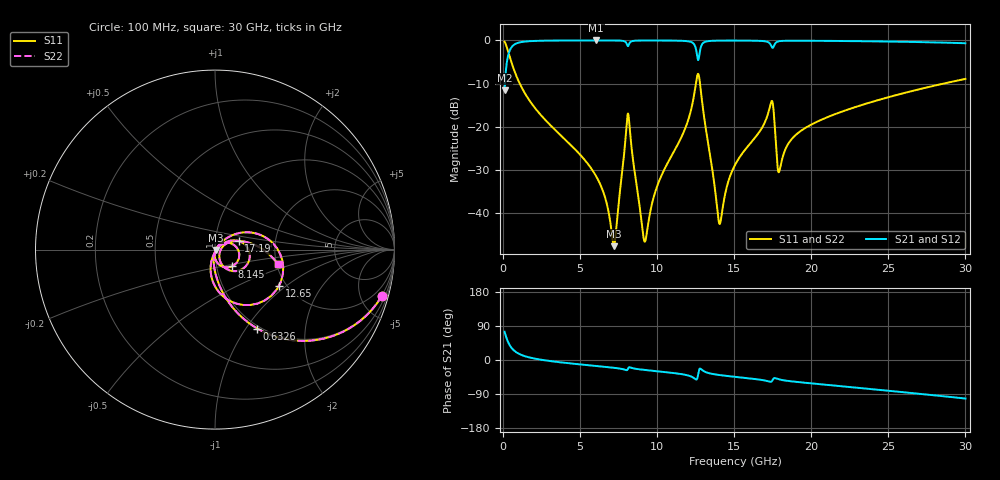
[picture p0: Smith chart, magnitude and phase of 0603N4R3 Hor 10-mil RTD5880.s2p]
# GHz S MA R 50
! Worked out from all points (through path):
!   3201 points, 100 MHz to 30 GHz, reference 50 ohm
!   highest |S21| = -0.03 dB at 6.043 GHz (marker M1); lowest = -11.6 dB at 100 MHz (marker M2)
!   group delay of S21, straight-line fit = 10.4 ps
!   lowest |S11| = -47.6 dB at 7.192 GHz (marker M3), VSWR 1.01, Z = 50.4 - j0.192 ohm
!   |S11| at or under -10 dB: 1.082 GHz to 12.51 GHz (11.43 GHz wide, 168 % of centre); 12.78 GHz to 28.58 GHz (15.8 GHz wide, 76.4 % of centre)
!   |S22| runs from -47.6 to -0.3 dB; largest |S21 - S12| = 0
!   S11 on the Smith chart (normalised r, x): 100 MHz: 0.97, -7.19; 632.6 MHz: 0.97, -1.13; 8.145 GHz: 1.19, -0.23; 12.65 GHz: 1.83, -0.89; 17.19 GHz: 1.30, +0.13; 30 GHz: 2.03, -0.37
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0.1  0.9646 -15.6  0.2635 74.4  0.2635 74.4  0.9646 -15.6
0.6325937  0.4988 -61.8  0.866 28.1  0.866 28.1  0.4988 -61.8
1.66975  0.207 -82.5  0.9771 7.1  0.9771 7.1  0.207 -82.5
5.089563  0.04575 -99.1  0.9965 -12.0  0.9965 -12.0  0.04575 -99.1
6.042625  0.02677 -100.0  0.9968 -15.8  0.9968 -15.8  0.02677 -100.0
7.191906  0.004168 -27.2  0.9958 -20.6  0.9958 -20.6  0.004168 -27.2
8.004812  0.09984 18.9  0.9279 -27.0  0.9279 -27.0  0.09984 18.9
8.144969  0.1333 -44.6  0.8771 -20.1  0.8771 -20.1  0.1333 -44.6
9.163438  0.004768 -33.7  0.9951 -26.1  0.9951 -26.1  0.004768 -33.7
10.06978  0.02226 48.5  0.9952 -30.0  0.9952 -30.0  0.02226 48.5
12.32162  0.1979 29.2  0.9308 -46.0  0.9308 -46.0  0.1979 29.2
12.64866  0.4099 -29.5  0.5942 -40.2  0.5942 -40.2  0.4099 -29.5
12.99437  0.1509 -97.7  0.9357 -28.7  0.9357 -28.7  0.1509 -97.7
14.02219  0.007683 -46.0  0.9922 -39.6  0.9922 -39.6  0.007683 -46.0
15.05  0.03618 36.4  0.9934 -44.5  0.9934 -44.5  0.03618 36.4
17.18972  0.1413 19.8  0.9557 -56.1  0.9557 -56.1  0.1413 19.8
17.47938  0.1948 -28.7  0.8198 -53.7  0.8198 -53.7  0.1948 -28.7
17.92788  0.03071 -7.0  0.9776 -51.4  0.9776 -51.4  0.03071 -7.0
18.638  0.06889 27.6  0.9897 -55.9  0.9897 -55.9  0.06889 27.6
20.03956  0.107 25.1  0.9882 -61.8  0.9882 -61.8  0.107 25.1
25.01978  0.2204 7.2  0.9688 -81.2  0.9688 -81.2  0.2204 7.2
30  0.3582 -12.8  0.9259 -101.7  0.9259 -101.7  0.3582 -12.8
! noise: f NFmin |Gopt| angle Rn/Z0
0.1  0.0003726  0.9364  0.7481  0.001306
3.417  0.003719  0.7955  9.968  0.00373
6.743  0.006905  0.785  19.35  0.006416
10.06  0.009843  0.7778  28.64  0.00852
13.39  0.02137  0.8591  37.92  0.02907
16.7  0.01879  0.8081  46.76  0.01721
20.03  0.01563  0.7379  55.39  0.00941
23.35  0.01713  0.7271  63.68  0.009095
26.67  0.01938  0.7286  71.76  0.009448
30  0.02191  0.7336  79.59  0.009847
